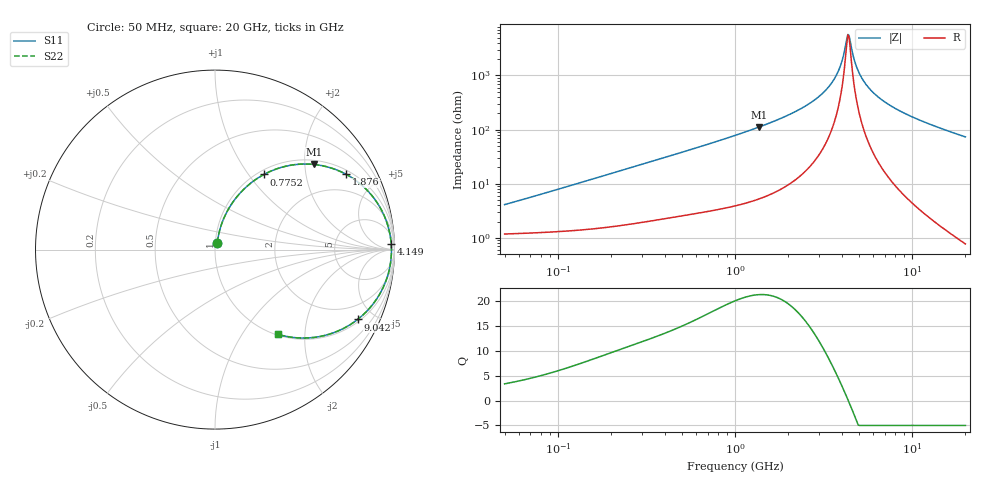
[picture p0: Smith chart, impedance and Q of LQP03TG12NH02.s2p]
!Murata Part Number: LQP03TG12NH02
!These Parameters are Measured in Series Mode Connection
!  o--[Z]--o
!Port1  Port2
!  o-------o
!Freq. Start=50[MHz] Stop=20[GHz], 401[Steps]
# Hz S RI R 50
!Freq.(Hz) S11(Real) S11(Imag) S21(Real) S21(Imag) S12(Real) S12(Imag) S22(Real) S22(Imag)
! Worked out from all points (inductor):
!   401 points, 50 MHz to 20 GHz, reference 50 ohm
!   read as one part in series: L = 12.5 nH near 51.52 MHz
!   highest Q = 21.3 at 1.37 GHz (marker M1), where L = 13 nH
!   self-resonance near 4.34 GHz
!   S11 on the Smith chart (normalised r, x): 50 MHz: 1.02, +0.08; 775.2 MHz: 1.07, +1.19; 1.876 GHz: 1.17, +3.38; 4.149 GHz: 28, +49; 9.042 GHz: 1.12, -4.02; 20 GHz: 1.02, -1.47
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5e7  0.0132 0.0385  0.9868 -0.0385  0.9868 -0.0385  0.0132 0.0385
1.364002e8  0.0245 0.1018  0.9755 -0.1018  0.9755 -0.1018  0.0245 0.1018
3.721004e8  0.0913 0.2522  0.9087 -0.2522  0.9087 -0.2522  0.0913 0.2522
7.751977e8  0.2724 0.4185  0.7276 -0.4185  0.7276 -0.4185  0.2724 0.4185
1e9  0.3843 0.4621  0.6157 -0.4621  0.6157 -0.4621  0.3843 0.4621
1.369645e9  0.5537 0.4741  0.4463 -0.4741  0.4463 -0.4741  0.5537 0.4741
1.875929e9  0.731 0.4192  0.269 -0.4192  0.269 -0.4192  0.731 0.4192
2.728004e9  0.8994 0.2674  0.1006 -0.2674  0.1006 -0.2674  0.8994 0.2674
3.168813e9  0.9433 0.1877  0.0567 -0.1877  0.0567 -0.1877  0.9433 0.1877
3.572216e9  0.9671 0.1192  0.0329 -0.1192  0.0329 -0.1192  0.9671 0.1192
3.908127e9  0.978 0.0661  0.022 -0.0661  0.022 -0.0661  0.978 0.0661
4.149438e9  0.9819 0.0301  0.0181 -0.0301  0.0181 -0.0301  0.9819 0.0301
4.275624e9  0.9829 0.0121  0.0171 -0.0121  0.0171 -0.0121  0.9829 0.0121
4.405649e9  0.9831 -0.00599  0.0169 0.00599  0.0169 0.00599  0.9831 -0.00599
4.472136e9  0.983 -0.015  0.017 0.015  0.017 0.015  0.983 -0.015
4.81993e9  0.9799 -0.0602  0.0201 0.0602  0.0201 0.0602  0.9799 -0.0602
5.273168e9  0.9707 -0.1138  0.0293 0.1138  0.0293 0.1138  0.9707 -0.1138
6.125241e9  0.9418 -0.2004  0.0582 0.2004  0.0582 0.2004  0.9418 -0.2004
7.442007e9  0.8804 -0.3034  0.1196 0.3034  0.1196 0.3034  0.8804 -0.3034
9.041845e9  0.7948 -0.3891  0.2052 0.3891  0.2052 0.3891  0.7948 -0.3891
1.334722e10  0.577 -0.4856  0.423 0.4856  0.423 0.4856  0.577 -0.4856
2e10  0.3509 -0.472  0.6491 0.472  0.6491 0.472  0.3509 -0.472
